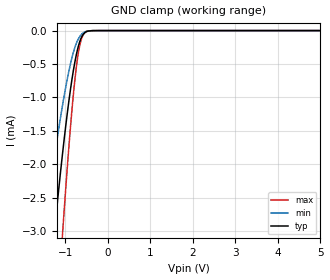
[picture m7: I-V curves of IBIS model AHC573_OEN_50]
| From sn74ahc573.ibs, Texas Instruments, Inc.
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[Model]   AHC573_OEN_50
Model_type  Input
Vinl=1.65
Vinh=3.85
| variable   typ   min   max
C_comp   0.76pF   0.69pF   0.92pF
[Temperature Range]   40   100   -40
| Ambient temperature   25   85   -40
[Voltage range]   5   4.5   5.5
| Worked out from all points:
|   GND clamp passes 1 mA (typ) near -0.91 V on its own axis
[GND Clamp]
| AHC573_OEN_50
|   Voltage   I(typ)   I(min)   I(max)
-5V       -39.31mA   -25.95mA   -50.22mA
-1.5V     -4.713mA   -3.013mA   -7.44mA
-1.27V    -3.094mA   -1.946mA   -5.018mA
-1.245V   -2.93mA    -1.837mA   -4.764mA
-1.07V    -1.855mA   -1.127mA   -3.064mA
-1.05V    -1.741mA   -1.053mA   -2.879mA
-875mV    -855.1uA   -482uA     -1.4mA
-765mV    -430.2uA   -230.3uA   -665uA
-665mV    -170.7uA   -92.19uA   -230.3uA
-615mV    -91.95uA   -52.35uA   -111.8uA
-545mV    -32.01uA   -20.16uA   -32.38uA
5V        14.69nA    957pA      135.7nA
